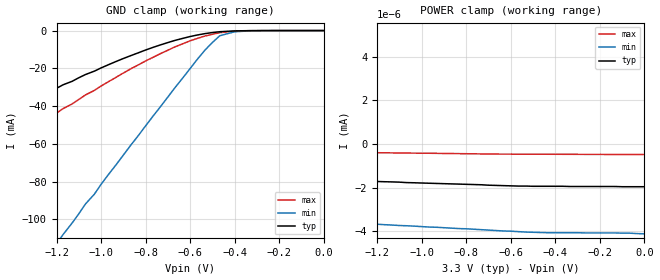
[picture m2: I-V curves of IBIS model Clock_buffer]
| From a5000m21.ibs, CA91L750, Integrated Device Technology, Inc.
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|   Model data
[Model]   Clock_buffer
Model_type   Input
Vinl =   1.33V
Vinh =   1.74V
C_comp   4.0000pF   3.5000pF   4.5000pF
[Temperature Range]   25.0000   80.0000   -40.0000
[Voltage Range]   3.3000V   3.0000V   3.6000V
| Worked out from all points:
|   GND clamp passes 1 mA (typ) near -0.50 V on its own axis
[GND_clamp]
|   voltage   I(typ)   I(min)   I(max)
-3.3V     -160mA     -433mA     -199mA
-2.43V    -107mA     -305mA     -137mA
-2.33V    -101mA     -290mA     -130mA
-2.03V    -81.7mA    -243mA     -107mA
-1.93V    -75.3mA    -228mA     -99.8mA
-1.17V    -28.7mA    -108mA     -41.3mA
-1.13V    -26.9mA    -102mA     -38.9mA
-733mV    -7.58mA    -40.3mA    -12.2mA
-533mV    -1.6mA     -10.3mA    -2.86mA
-467mV    -610uA     -2.77mA    -1.12mA
-333mV    -45.1uA    -162uA     -58.5uA
0V        -149pA     -121pA     -77.8pA
[POWER_clamp]
|   voltage   I(typ)   I(min)   I(max)
-3.3V     93nA       18.7mA     44.8nA
-3.27V    -693pA     13.5mA     -165pA
-3.2V     -1.01nA    4.63mA     -174pA
-2.77V    -1.23nA    6.06nA     -219pA
-2.73V    -1.24nA    -442pA     -222pA
-2.7V     -1.25nA    -1.92nA    -226pA
-2.67V    -1.26nA    -2.58nA    -230pA
-2.63V    -1.27nA    -2.73nA    -234pA
-2.37V    -1.36nA    -3.03nA    -264pA
-1.47V    -1.64nA    -3.55nA    -368pA
-533mV    -1.93nA    -4.04nA    -467pA
0V        -1.96nA    -4.12nA    -483pA
